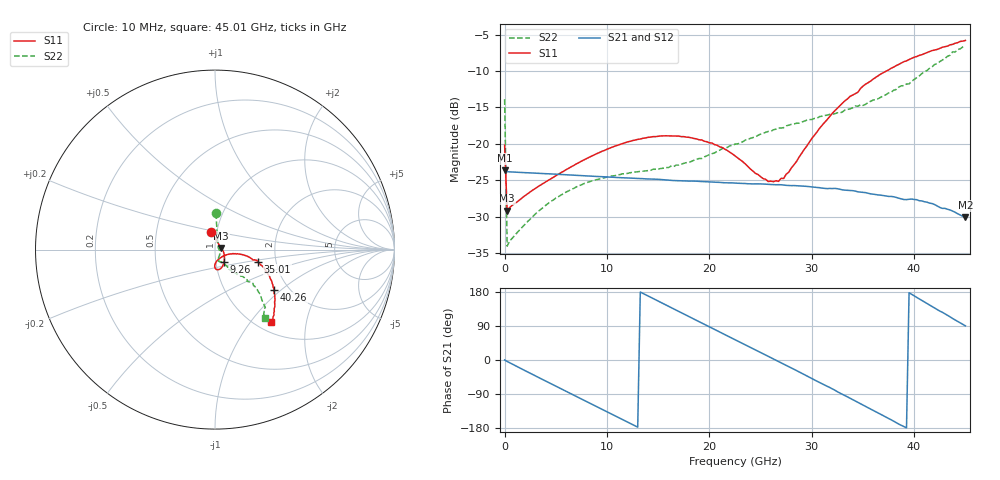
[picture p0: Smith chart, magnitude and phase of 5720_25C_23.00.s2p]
! Device:  ADRF5720
! Description: 0.5dB LSB GaAs MMIC 6-bit Digital Attenuator
! Frequency:  0.000009 -  40 GHz
! Ports:
!	RF1	= Port 1
!	RF2	= Port 2
! Vdd:  3.3 Volt
! Vss:  -3.3 Volt
! Control:  0/3.3 Volt
! State:  23.00 dB attenuation
! Data:  The device was measured using G-S-G Probes on a matrix board.
!  Data was collected using an calibrated 4 port network analyzer.
!  The reference plane for this measurement is at the launchers.
! Note:  Analog Devices supplies this data as a sample of measured data
!  for this product.  Your particular data for this product may vary.
!  Data was taken at 25 degrees C.
!  Analog Devices reserves the right to change this data at anytime.
# GHZ S DB R 45.0
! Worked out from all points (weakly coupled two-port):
!   181 points, 10 MHz to 45.01 GHz, reference 45 ohm
!   highest |S21| = -23.64 dB at 10 MHz (marker M1); lowest = -30.1 dB at 45.01 GHz (marker M2)
!   lowest |S11| = -29.2 dB at 260 MHz (marker M3), VSWR 1.07, Z = 48.1 + j0.872 ohm
!   |S11| at or under -10 dB: start of sweep to 37.3 GHz
!   |S22| runs from -34.0 to -6.6 dB; largest |S21 - S12| = 0.00013
!   S11 on the Smith chart (normalised r, x): 10 MHz: 0.94, +0.18; 9.26 GHz: 1.09, -0.16; 35.01 GHz: 1.61, -0.23; 40.26 GHz: 1.67, -0.90; 45.01 GHz: 1.16, -1.28
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0.01  -20.18 102.0  -23.64 0.1  -23.63 0.1  -13.88 88.7
0.26  -29.19 15.1  -23.83 -3.8  -23.83 -3.8  -34.05 24.6
1.26  -27.95 0.1  -23.90 -17.8  -23.90 -17.8  -32.15 -7.3
3.51  -25.67 -19.8  -24.06 -48.6  -24.06 -48.6  -29.03 -40.9
5.01  -24.38 -31.1  -24.17 -69.0  -24.17 -69.0  -27.45 -55.1
7.76  -22.20 -47.3  -24.38 -106.2  -24.38 -106.2  -25.46 -69.8
9.26  -21.20 -54.6  -24.49 -126.5  -24.49 -126.5  -24.83 -74.1
12.01  -19.74 -66.5  -24.69 -163.7  -24.69 -163.7  -24.06 -76.9
15.26  -18.92 -78.1  -24.90 151.8  -24.90 151.9  -23.39 -73.2
19.26  -19.47 -88.7  -25.18 97.7  -25.18 97.7  -22.02 -62.6
21.26  -20.51 -90.8  -25.32 70.5  -25.32 70.5  -20.67 -58.4
22.76  -21.93 -89.7  -25.41 50.3  -25.41 50.3  -20.01 -55.8
25.76  -25.18 -62.9  -25.56 9.7  -25.56 9.7  -18.30 -54.0
26.76  -25.15 -46.0  -25.61 -3.9  -25.62 -3.9  -17.82 -53.0
27.76  -23.89 -29.0  -25.72 -17.6  -25.72 -17.6  -17.44 -53.1
30.26  -18.82 -11.4  -25.95 -52.2  -25.95 -52.2  -16.52 -52.5
32.26  -15.45 -10.9  -26.12 -79.7  -26.11 -79.6  -15.88 -50.8
35.01  -12.08 -15.9  -26.67 -118.8  -26.68 -118.8  -14.73 -47.9
37.76  -9.63 -25.3  -27.22 -157.7  -27.23 -157.7  -12.92 -43.6
40.26  -8.01 -34.5  -27.67 165.2  -27.67 165.2  -10.92 -41.7
43.76  -6.35 -47.1  -29.23 109.5  -29.23 109.5  -7.37 -49.0
45.01  -5.81 -52.1  -30.09 90.2  -30.12 90.3  -6.55 -53.7
